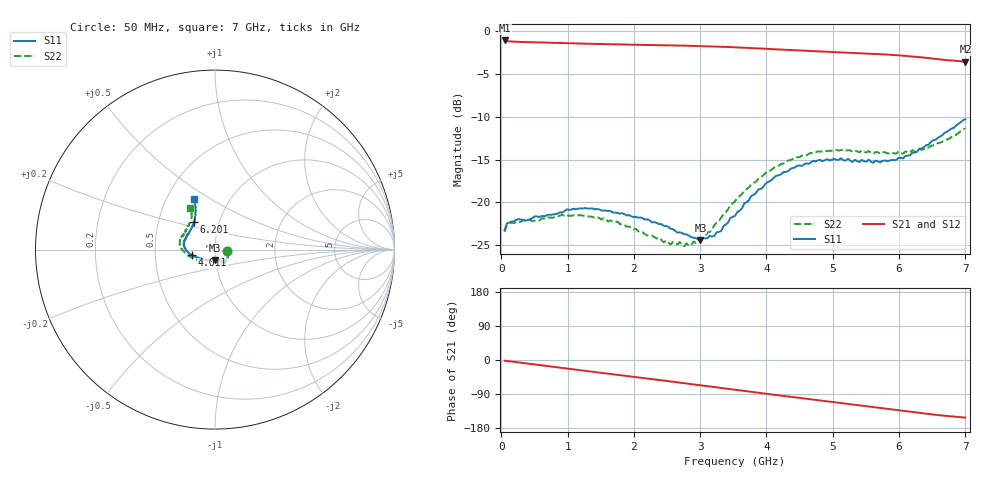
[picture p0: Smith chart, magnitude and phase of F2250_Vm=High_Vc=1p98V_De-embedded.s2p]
! Integrated Device Technology
! Corporate Headquarters
! 6024 Silver Creek Valley Road
! San Jose, CA 95138  USA
! Phone:  1-408-284-8200
! Toll Free:  1-800-223-1366
! Webpage:  http://www.idt.com/
! Timing and RF Division
! 515 Groton Road, Suite 102
! Westford, MA 01886-6024
! Device:  F2250
! Description: Voltage Variable RF Attenuator
! Frequency:  50.0 -  6000.00 MHz
! Package:  3x3 mm Thin QFN Plastic Package: 16 pin
! Ports:  2 RF, 3 DC
!  Pin  1  = GND
!  Pin  2  = NC
!  Pin  3  = RF1  = Port 1
!  Pin  4  = NC
!  Pin  5  = GND
!  Pin  6  = GND
!  Pin  7  = GND
!  Pin  8  = GND
!  Pin  9  = NC
!  Pin 10  = RF2  = Port 2
!  Pin 11  = NC
!  Pin 12  = GND
!  Pin 13  = GND
!  Pin 14  = VCNTRL
!  Pin 15  = VDD
!  Pin 16  = VMODE
! Vcntrl:  1.980 Volts
! Vmode:  +3.300 Volts
! Vdd:  +3.30  Volts
! Current:  1.324 mA
! Data:  The device was measured on a the F2250 evaluation board which has
!  individual transmission lines to the RF pins.  Data was collected
!  using a calibrated network analyzer.  The evaluation board was
!  de-embedded using a TRL calibration technique.
!  The reference plane is the edge of the package pin.
! Misc:  SN 10
!  Action Tracker AT0258
! Date Measured:  2014-11-26
! Date:  2015-10-15  MJV
! Note:
!  Integrated Device Technology supplies this data as a sample of measured
!  data at the package pin for this product.  Your particular data for this
!  product may vary.
!  Data was taken at 25 degrees C.
!  Integrated Device Technology reserves the right to change this data at anytime.
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# GHz S dB R 50
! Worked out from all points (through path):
!   201 points, 50 MHz to 7 GHz, reference 50 ohm
!   highest |S21| = -1.05 dB at 50 MHz (marker M1); lowest = -3.5 dB at 7 GHz (marker M2)
!   group delay of S21, straight-line fit = 61.1 ps
!   lowest |S11| = -24.4 dB at 3.004 GHz (marker M3), VSWR 1.13, Z = 49.5 - j5.97 ohm
!   |S11| at or under -10 dB: start of sweep to end of sweep
!   |S22| runs from -25.2 to -11.4 dB; largest |S21 - S12| = 0.0018
!   S11 on the Smith chart (normalised r, x): 50 MHz: 1.15, -0.02; 4.011 GHz: 0.77, -0.05; 6.201 GHz: 0.76, +0.24; 7 GHz: 0.68, +0.42
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0.05  -23.26 -8.3  -1.05 -1.8  -1.05 -1.8  -23.48 -9.0
0.08475  -22.49 -7.6  -1.13 -2.5  -1.13 -2.5  -22.62 -8.1
0.1195  -22.37 -8.2  -1.16 -3.3  -1.16 -3.3  -22.43 -7.7
0.91875  -21.23 -42.9  -1.35 -21.1  -1.35 -21.1  -21.48 -46.6
1.2315  -20.74 -50.6  -1.42 -27.9  -1.42 -27.9  -21.58 -57.0
1.75275  -21.25 -57.5  -1.51 -39.1  -1.51 -39.1  -22.28 -65.3
2.37825  -22.57 -58.6  -1.60 -52.7  -1.61 -52.7  -24.20 -70.1
2.44775  -22.76 -60.6  -1.61 -54.3  -1.61 -54.3  -24.71 -73.0
2.691  -23.53 -69.0  -1.65 -59.7  -1.65 -59.7  -24.66 -83.4
2.7605  -23.74 -70.7  -1.66 -61.2  -1.66 -61.2  -25.15 -87.4
3.00375  -24.43 -91.0  -1.71 -66.7  -1.71 -66.7  -24.23 -108.2
3.21225  -23.96 -112.1  -1.76 -71.4  -1.75 -71.4  -22.70 -126.0
3.525  -21.61 -140.5  -1.85 -78.5  -1.85 -78.5  -19.89 -144.9
3.76825  -19.28 -155.8  -1.94 -84.0  -1.94 -84.0  -17.93 -156.4
4.0115  -17.66 -165.8  -2.04 -89.4  -2.04 -89.4  -16.37 -166.3
4.4285  -15.94 -178.3  -2.20 -98.6  -2.21 -98.6  -14.75 -179.2
4.7065  -15.17 174.3  -2.30 -104.8  -2.30 -104.8  -14.27 174.8
5.054  -15.04 165.9  -2.43 -112.4  -2.42 -112.5  -13.88 167.4
5.85325  -15.15 139.4  -2.73 -129.9  -2.73 -130.0  -14.28 148.3
6.20075  -14.19 127.0  -2.93 -137.6  -2.93 -137.7  -13.91 139.1
6.54825  -12.68 118.4  -3.20 -144.6  -3.20 -144.8  -13.30 127.7
7  -10.29 113.0  -3.53 -152.0  -3.54 -152.1  -11.35 121.2
